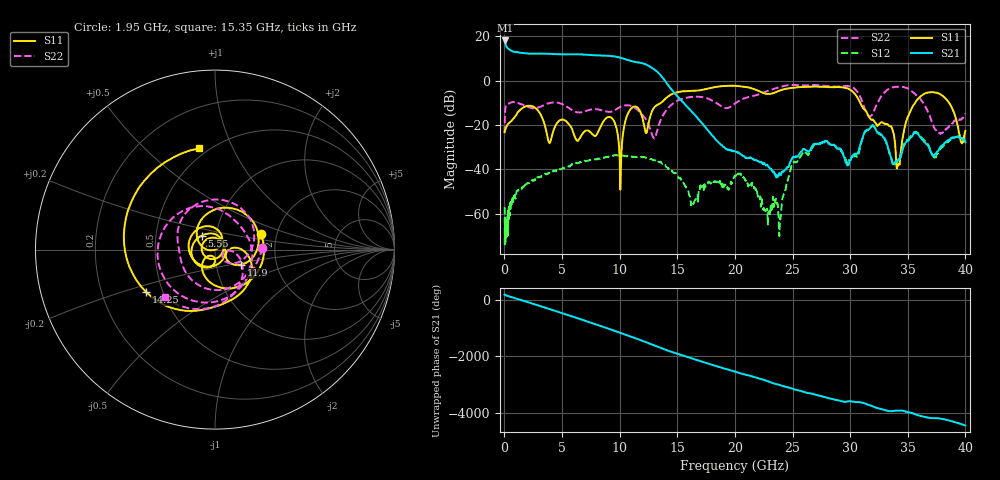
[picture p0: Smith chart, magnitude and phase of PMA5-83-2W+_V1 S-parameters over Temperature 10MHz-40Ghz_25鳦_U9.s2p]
!Mini-Circuits Laboratory
!S-Parameters
!Model: US-AMP-1
!Run / Lot / Date Code: N/A / N/A / N/A
!Fixture: N/A, Pressing Arm: N/A
!Network Analyzer: NFA N8975A;  Serial number: 74408
!Date: 11/29/2023 at 9:46:45 AM
!No.: Unit# 2 (U9)
!Tested with: +25°C
! 2 port cal with Bias Tee PE1622 in line. No normalization applied. Bias cond 2: Vdd= 12V, Idd= 400mA, Vg2= 5V, starting point for Vg1= -2V
# Hz  S  dB  R  50
!Frequency  S11 dB  S11 Deg  S21 dB  S21 Deg  S12 dB  S12 Deg  S22 dB  S22 Deg
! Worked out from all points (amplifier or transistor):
!   826 points, 10 MHz to 40 GHz, reference 50 ohm
!   highest |S21| = 18.2 dB at 20 MHz (marker M1)
!   |S21| within 3 dB of that: start of sweep to 192.6 MHz
!   unconditionally stable (mu >= 1): start of sweep to end of sweep
!   at 5.6 GHz: K = 9.88, MAG = 12.3 dB, |S12| = -38.5 dB
!   at 19.4 GHz: K = 1834.77, MAG = -26.9 dB, |S12| = -48.5 dB
!   at 40 GHz: K = 272.28, MAG = -27.6 dB, |S12| = -27.3 dB
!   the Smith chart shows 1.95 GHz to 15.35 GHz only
!   S11 on the Smith chart (normalised r, x): 1.95 GHz: 1.65, +0.31; 5.55 GHz: 0.86, +0.14; 11.9 GHz: 1.31, -0.23; 14.25 GHz: 0.40, -0.24; 15.35 GHz: 0.45, +0.75
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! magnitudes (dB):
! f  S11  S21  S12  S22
! 10 MHz  -23.0  18.0  -57.1  -23.8
! 20 MHz  -22.9  18.2  -60.4  -19.8
! 1.95 GHz  -11.4  12.3  -46.3  -11.6
! 5.55 GHz  -19.5  11.9  -38.6  -12.2
! 6.7 GHz  -24.5  11.9  -36.7  -14.2
! 9.2 GHz  -16.5  11.2  -34.1  -14.1
! 10.05 GHz  -49.1  10.4  -33.6  -11.8
! 10.8 GHz  -13.9  9.2  -34.0  -11.1
! 11.9 GHz  -15.5  8.0  -34.4  -15.0
! 13.35 GHz  -10.6  3.6  -36.6  -20.8
! 14.25 GHz  -6.9  -2.3  -39.6  -12.1
! 15.35 GHz  -4.9  -9.0  -45.0  -8.3
! 20.05 GHz  -2.3  -32.0  -43.2  -10.1
! 23.85 GHz  -4.5  -41.7  -70.1  -2.9
! 26.7 GHz  -2.6  -29.6  -30.3  -1.9
! 29.8 GHz  -3.5  -37.8  -37.1  -2.4
! 31.7 GHz  -16.9  -21.6  -21.7  -16.1
! 33.35 GHz  -20.3  -31.4  -31.5  -3.7
! 34.2 GHz  -37.4  -35.3  -35.9  -2.7
! 35.3 GHz  -12.8  -25.4  -24.9  -4.6
! 37.2 GHz  -5.2  -34.0  -33.9  -20.1
! 40 GHz  -22.6  -27.7  -27.3  -14.9
